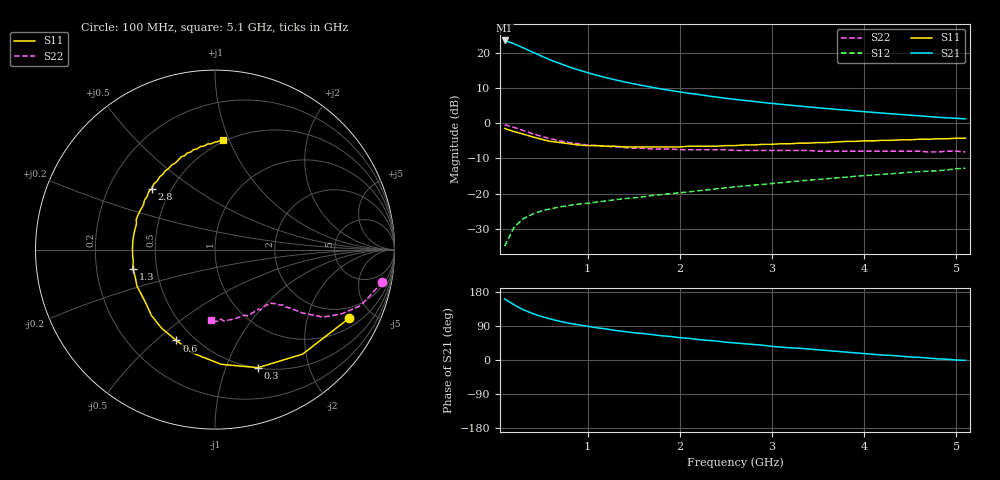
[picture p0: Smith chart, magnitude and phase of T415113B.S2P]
!AT-41511
!S-PARAMETERS at Vce=2.7V  Ic=5mA.  LAST UPDATED 01-25-95
# ghz s ma r 50
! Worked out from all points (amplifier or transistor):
!   51 points, 100 MHz to 5.1 GHz, reference 50 ohm
!   highest |S21| = 23.4 dB at 100 MHz (marker M1)
!   |S21| within 3 dB of that: start of sweep to 379.2 MHz
!   unconditionally stable (mu >= 1): 1.585 GHz to 4.525 GHz; 4.64 GHz to 4.829 GHz
!   at 900 MHz: K = 0.72, MSG = 19.0 dB, |S12| = -23.0 dB
!   at 2.6 GHz: K = 1.12, MAG = 10.3 dB, |S12| = -18.1 dB
!   at 5.1 GHz: K = 0.96, MSG = 7.0 dB, |S12| = -12.8 dB
!   lowest NFmin = 0.80 dB at 100 MHz
!   S11 on the Smith chart (normalised r, x): 100 MHz: 1.41, -3.65; 300 MHz: 0.50, -1.30; 600 MHz: 0.40, -0.58; 1.3 GHz: 0.36, -0.10; 2.8 GHz: 0.39, +0.35; 5.1 GHz: 0.49, +0.95
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0.1  0.84 -27.0  14.85 161.0  0.018 76.0  0.95 -11.0
0.2  0.76 -50.0  13.38 146.0  0.033 65.0  0.87 -21.0
0.3  0.7 -70.0  11.72 133.0  0.044 57.0  0.79 -27.0
0.4  0.64 -87.0  10.22 123.0  0.051 52.0  0.71 -32.0
0.5  0.59 -102.0  8.924 115.0  0.057 48.0  0.65 -34.0
0.6  0.55 -113.0  7.828 108.0  0.061 46.0  0.6 -36.0
0.7  0.53 -124.0  6.993 102.0  0.065 44.0  0.56 -37.0
0.8  0.51 -134.0  6.275 97.0  0.068 43.0  0.53 -38.0
0.9  0.49 -141.0  5.684 93.0  0.071 43.0  0.51 -39.0
1  0.48 -149.0  5.189 89.0  0.073 43.0  0.49 -39.0
1.1  0.48 -155.0  4.767 85.0  0.076 43.0  0.48 -40.0
1.3  0.47 -167.0  4.107 78.0  0.082 43.0  0.46 -41.0
1.5  0.46 -176.0  3.61 72.0  0.087 44.0  0.44 -43.0
1.8  0.46 170.0  3.051 64.0  0.097 45.0  0.43 -45.0
2.2  0.47 155.0  2.548 54.0  0.11 46.0  0.42 -49.0
2.6  0.48 142.0  2.174 45.0  0.125 46.0  0.41 -54.0
2.8  0.49 136.0  2.035 41.0  0.132 45.0  0.41 -56.0
3.1  0.51 127.0  1.846 34.0  0.143 45.0  0.41 -60.0
3.5  0.53 117.0  1.649 27.0  0.159 44.0  0.4 -66.0
4  0.56 106.0  1.454 17.0  0.18 42.0  0.4 -73.0
4.3  0.57 100.0  1.355 12.0  0.192 40.0  0.4 -78.0
5.1  0.61 86.0  1.149 -1.0  0.23 36.0  0.39 -93.0
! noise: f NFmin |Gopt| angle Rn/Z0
0.1  0.8  0.45  6  0.25
0.9  1  0.39  63  0.19
1.8  1.4  0.32  137  0.12
2.4  1.7  0.4  177  0.09
